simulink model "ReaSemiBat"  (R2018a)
settings: Solver=VariableStepAuto  StartTime=0.0  StopTime=150  RelTol=1e-3
undefined symbols (not defined in the file): a0fd, a12a, a4d45f35, b078, d7f8158e, db7ea239839c, fb44, ReaSemiBat, sdiscope

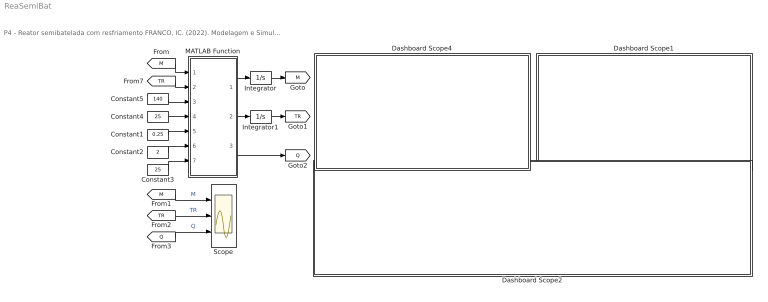
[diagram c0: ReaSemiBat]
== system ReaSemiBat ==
  note: P4 - Reator semibatelada com resfriamento FRANCO, IC. (2022). Modelagem e Simulação: Problemas Típicos da Engenharia Química para Simulação e Análise. NOTAS DE AULA INOVADORAS. The Journal of Engineering and Exact Sciences. Material Complementar.
  Constant1 : Constant  Value=0.25
  Constant2 : Constant  Value=2
  Constant3 : Constant  Value=25
  Constant4 : Constant  Value=25
  Constant5 : Constant  Value=140
  Dashboard Scope1 : Subsystem  DialogController=hmiCreateDDGDialog  IsWebBlock=on  mask(MWDashboardBlock){webBlockId=d7f8158e-0b85-46ef-b078-374dc6de96e0, webBlockType=sdiscope, ShowInitialText=on, HMISrcModelName=ReaSemiBat}
      mask prompts: webBlockId "WebBlock Id"; webBlockType "WebBlock Type"; HMISrcModelName "Source Model"
      mask help: SimulinkHMI:dialogs:HMIScopeDialogDesc
  Dashboard Scope2 : Subsystem  DialogController=hmiCreateDDGDialog  IsWebBlock=on  mask(MWDashboardBlock){webBlockId=5cfab876-fb44-4ffb-a12a-969179e93a1c, webBlockType=sdiscope, ShowInitialText=on, HMISrcModelName=ReaSemiBat}
      mask prompts: webBlockId "WebBlock Id"; webBlockType "WebBlock Type"; HMISrcModelName "Source Model"
      mask help: SimulinkHMI:dialogs:HMIScopeDialogDesc
  Dashboard Scope4 : Subsystem  DialogController=hmiCreateDDGDialog  IsWebBlock=on  mask(MWDashboardBlock){webBlockId=a4d45f35-6ac9-4911-a0fd-db7ea239839c, webBlockType=sdiscope, ShowInitialText=on, HMISrcModelName=ReaSemiBat}
      mask prompts: webBlockId "WebBlock Id"; webBlockType "WebBlock Type"; HMISrcModelName "Source Model"
      mask help: SimulinkHMI:dialogs:HMIScopeDialogDesc
  Integrator : Integrator  InitialCondition=1000
  Integrator1 : Integrator  InitialCondition=25
  MATLAB Function : MATLAB Function  TreatAsAtomicUnit=on
  Scope : Scope  NumInputPorts=3
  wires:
  Integrator/1 -> [M]
  [M] -> MATLAB Function/1(M)
  MATLAB Function/1(dM) -> Integrator/1
  MATLAB Function/3(Q) -> [Q]
  Integrator1/1 -> [TR]
  MATLAB Function/2(dTR) -> Integrator1/1
  Constant3/1 -> MATLAB Function/7(Tc)
  Constant2/1 -> MATLAB Function/6(A)
  Constant1/1 -> MATLAB Function/5(x0)
  Constant4/1 -> MATLAB Function/4(Ti)
  Constant5/1 -> MATLAB Function/3(W)
  [TR] -> MATLAB Function/2(TR)
  [Q] -> Scope/3  "Q"
  [TR] -> Scope/2  "TR"
  [M] -> Scope/1  "M"

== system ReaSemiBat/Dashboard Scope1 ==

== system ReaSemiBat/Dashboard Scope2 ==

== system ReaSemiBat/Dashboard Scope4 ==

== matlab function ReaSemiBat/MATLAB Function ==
function [dM,dTR,Q] = fcn(M,TR,W,Ti,x0,A,Tc)
%% Parâmetros
Cp  =    1.00;
U   =  415.00;
dH  =-1100.00;

%% condicional para mudança de semibatelada para batelada
if M>10000
   W=0;
end

%% Equações auxiliares;
Q = U*A*(TR-Tc)

%% Modelo matemático
dM  = W;
dTR = (W*Cp*(Ti-TR)+W*x0*(-dH)-Q)/(M*Cp);
end
